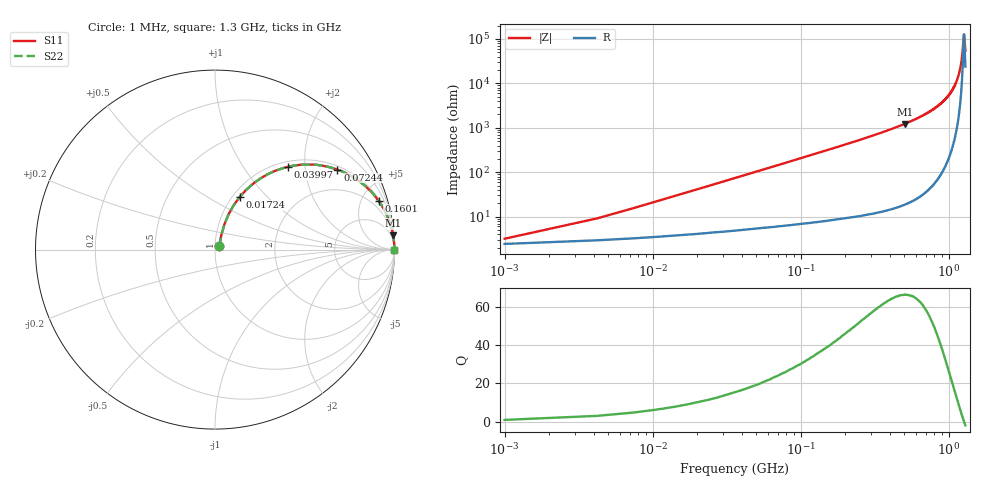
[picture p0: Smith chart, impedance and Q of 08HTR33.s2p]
! Coilcraft 0805HT-R33 Chip Inductor
! 6 August 2004
# MHZ S MA R 50
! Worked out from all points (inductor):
!   401 points, 1 MHz to 1.3 GHz, reference 50 ohm
!   read as one part in series: L = 326 nH near 7.495 MHz
!   highest Q = 66.2 at 507.6 MHz (marker M1), where L = 385 nH
!   self-resonance near 1.271 GHz
!   S11 on the Smith chart (normalised r, x): 1 MHz: 1.05, +0.04; 17.24 MHz: 1.08, +0.71; 39.97 MHz: 1.10, +1.64; 72.44 MHz: 1.12, +2.98; 160.1 MHz: 1.17, +6.66; 1.3 GHz: open
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1  0.031 39.2  0.976 -1.1  0.976 -1.1  0.031 39.2
10.743  0.211 68.9  0.945 -12.0  0.945 -12.0  0.211 68.9
17.238  0.324 64.9  0.911 -18.8  0.911 -18.8  0.324 64.9
26.98  0.469 57.5  0.846 -27.9  0.846 -27.9  0.469 57.5
39.97  0.616 48.5  0.751 -38.0  0.751 -38.0  0.616 48.5
72.445  0.815 33.1  0.547 -54.5  0.547 -54.5  0.815 33.1
108.168  0.902 23.8  0.404 -64.4  0.404 -64.4  0.902 23.8
160.128  0.951 16.6  0.285 -72.0  0.285 -72.0  0.951 16.6
218.583  0.973 12.2  0.211 -76.6  0.211 -76.6  0.973 12.2
436.165  0.994 5.6  0.098 -83.5  0.098 -83.5  0.994 5.6
507.61  0.996 4.6  0.081 -84.5  0.081 -84.5  0.996 4.6
650.5  0.998 3.2  0.055 -85.9  0.055 -85.9  0.998 3.2
868.082  0.999 1.7  0.03 -86.9  0.03 -86.9  0.999 1.7
1007.725  0.999 1.0  0.018 -86.7  0.018 -86.7  0.999 1.0
1085.665  0.999 0.7  0.012 -86.0  0.012 -86.0  0.999 0.7
1153.862  0.999 0.4  0.007544 -84.0  0.007544 -84.0  0.999 0.4
1202.575  0.999 0.2  0.004393 -79.9  0.004393 -79.9  0.999 0.2
1235.05  0.999 0.1  0.002409 -71.3  0.002409 -71.3  0.999 0.1
1264.277  0.999 0.0  0.0009214 -32.2  0.0009214 -32.2  0.999 0.0
1270.772  0.999 0.0  0.0007894 -7.1  0.0007894 -7.1  0.999 0.0
1277.267  0.999 -0.0  0.0008395 20.4  0.0008395 20.4  0.999 -0.0
1300  0.999 -0.1  0.001829 64.0  0.001829 64.0  0.999 -0.1
